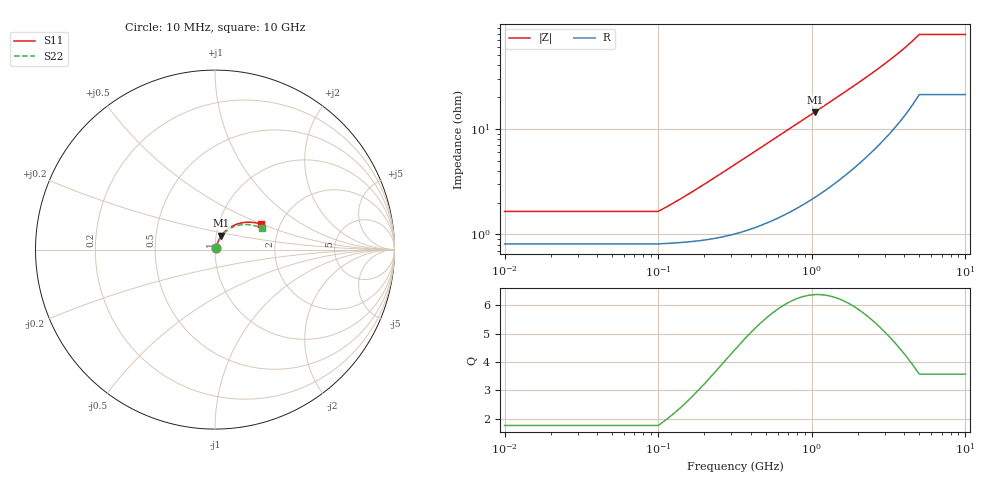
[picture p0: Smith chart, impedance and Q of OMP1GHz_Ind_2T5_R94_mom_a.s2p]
! Created Fri Jun 17 13:51:10 2016
# ghz S ma R 50
! 2 Port Network Data from SP1.SP block
! freq  magS11  angS11  magS21  angS21  magS12  angS12  magS22  angS22
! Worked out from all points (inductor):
!   1000 points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, 10 MHz to 10 GHz, reference 50 ohm
!   read as 1/Y11, port 2 shorted: L = 2.26 nH near 190 MHz
!   highest Q = 6.37 at 1.05 GHz (marker M1), where L = 2.17 nH
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0.01  0.01201 46.9  0.9919 -1.1  0.9919 -1.1  0.01202 46.8
0.06  0.01201 46.9  0.9919 -1.1  0.9919 -1.1  0.01202 46.8
0.1  0.01201 46.9  0.9919 -1.1  0.9919 -1.1  0.01202 46.8
0.13  0.01419 53.2  0.9917 -1.5  0.9917 -1.5  0.0142 53.0
0.22  0.02135 63.0  0.9909 -2.5  0.9909 -2.5  0.02136 62.8
0.28  0.02629 65.9  0.9901 -3.1  0.9901 -3.1  0.02631 65.5
0.37  0.03368 67.9  0.9888 -4.1  0.9888 -4.1  0.0337 67.4
0.48  0.04256 68.6  0.9869 -5.3  0.9869 -5.3  0.04258 68.1
0.6  0.05201 68.6  0.9846 -6.6  0.9846 -6.6  0.05202 67.8
0.73  0.06198 68.0  0.9819 -7.9  0.9819 -7.9  0.06198 67.1
0.88  0.07317 66.9  0.9786 -9.5  0.9786 -9.5  0.07315 65.9
1.05  0.08548 65.5  0.9745 -11.2  0.9745 -11.2  0.08543 64.2
1.34  0.1056 62.7  0.967 -14.1  0.967 -14.1  0.1055 61.2
1.68  0.1279 59.3  0.9573 -17.4  0.9573 -17.4  0.1277 57.4
2.02  0.1489 55.9  0.947 -20.7  0.947 -20.7  0.1486 53.6
2.41  0.1716 52.1  0.9346 -24.3  0.9346 -24.3  0.171 49.4
3.34  0.2201 43.3  0.9036 -32.6  0.9036 -32.6  0.2187 39.7
4.19  0.2589 35.8  0.8748 -39.9  0.8748 -39.9  0.2565 31.4
5.01  0.2922 29.1  0.8476 -46.6  0.8476 -46.6  0.2887 24.1
6.67  0.2922 29.1  0.8476 -46.6  0.8476 -46.6  0.2887 24.1
8.34  0.2922 29.1  0.8476 -46.6  0.8476 -46.6  0.2887 24.1
10  0.2922 29.1  0.8476 -46.6  0.8476 -46.6  0.2887 24.1
